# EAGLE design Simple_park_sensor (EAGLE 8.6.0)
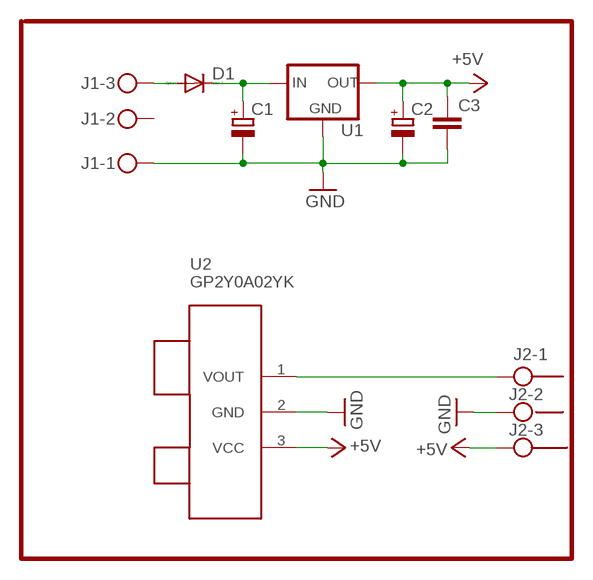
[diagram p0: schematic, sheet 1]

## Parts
C1  CPOL-EUC/6032-28W  [C/6032-28W]
C2  CPOL-EUC/6032-28W  [C/6032-28W]
C3  C-EUC1206  [C1206]
D1  CGRM4002-G  [SOD-123_MINI-SMA]
J1  MKDSN1,5/3-5,08  [MKDSN1,5/3-5,08]
J2  MKDSN1,5/3-5,08  [MKDSN1,5/3-5,08]
U1  78XXL  [78XXL]
U2  GP2Y0A02YK  [GP2Y0A02YK]

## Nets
+5V: C2.+ C3.1 J2.3 U1.OUT U2.3(VCC)
GND: C1.- C2.- C3.2 J1.1 J2.2 U1.GND U2.2(GND)
N$1: C1.+ D1.C U1.IN
N$2: D1.A J1.3
N$3: J2.1 U2.1(VOUT)
Unconnected: J1.2

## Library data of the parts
C1 C2 = rcl:CPOL-EU: POLARIZED CAPACITOR, European symbol
C3 = rcl:C-EU: CAPACITOR, European symbol
D1 = diode:CGRM400*-G: Molded plasitc,JEDEC SOD-123/Mini SMA
J1 J2 = con-phoenix-508:MKDSN1,5/3-5,08: MKDSN 1,5/ 3-5,08 Printklemme Nennstrom: 13,5 A Nennspannung: 250 V Rastermaß: 5,08 mm Polzahl: 3 Anschlussart: Schraubanschluss Montage: Löten Anschlussrichtung Leiter/Platine: 0 ° Artikelnummer: 1729131 Source: http://eshop.phoenixcontact.com .. 1729131.pdf
U1 = v-reg:78XXL: VOLTAGE REGULATOR
U2 = sharp:GP2Y0A02YK

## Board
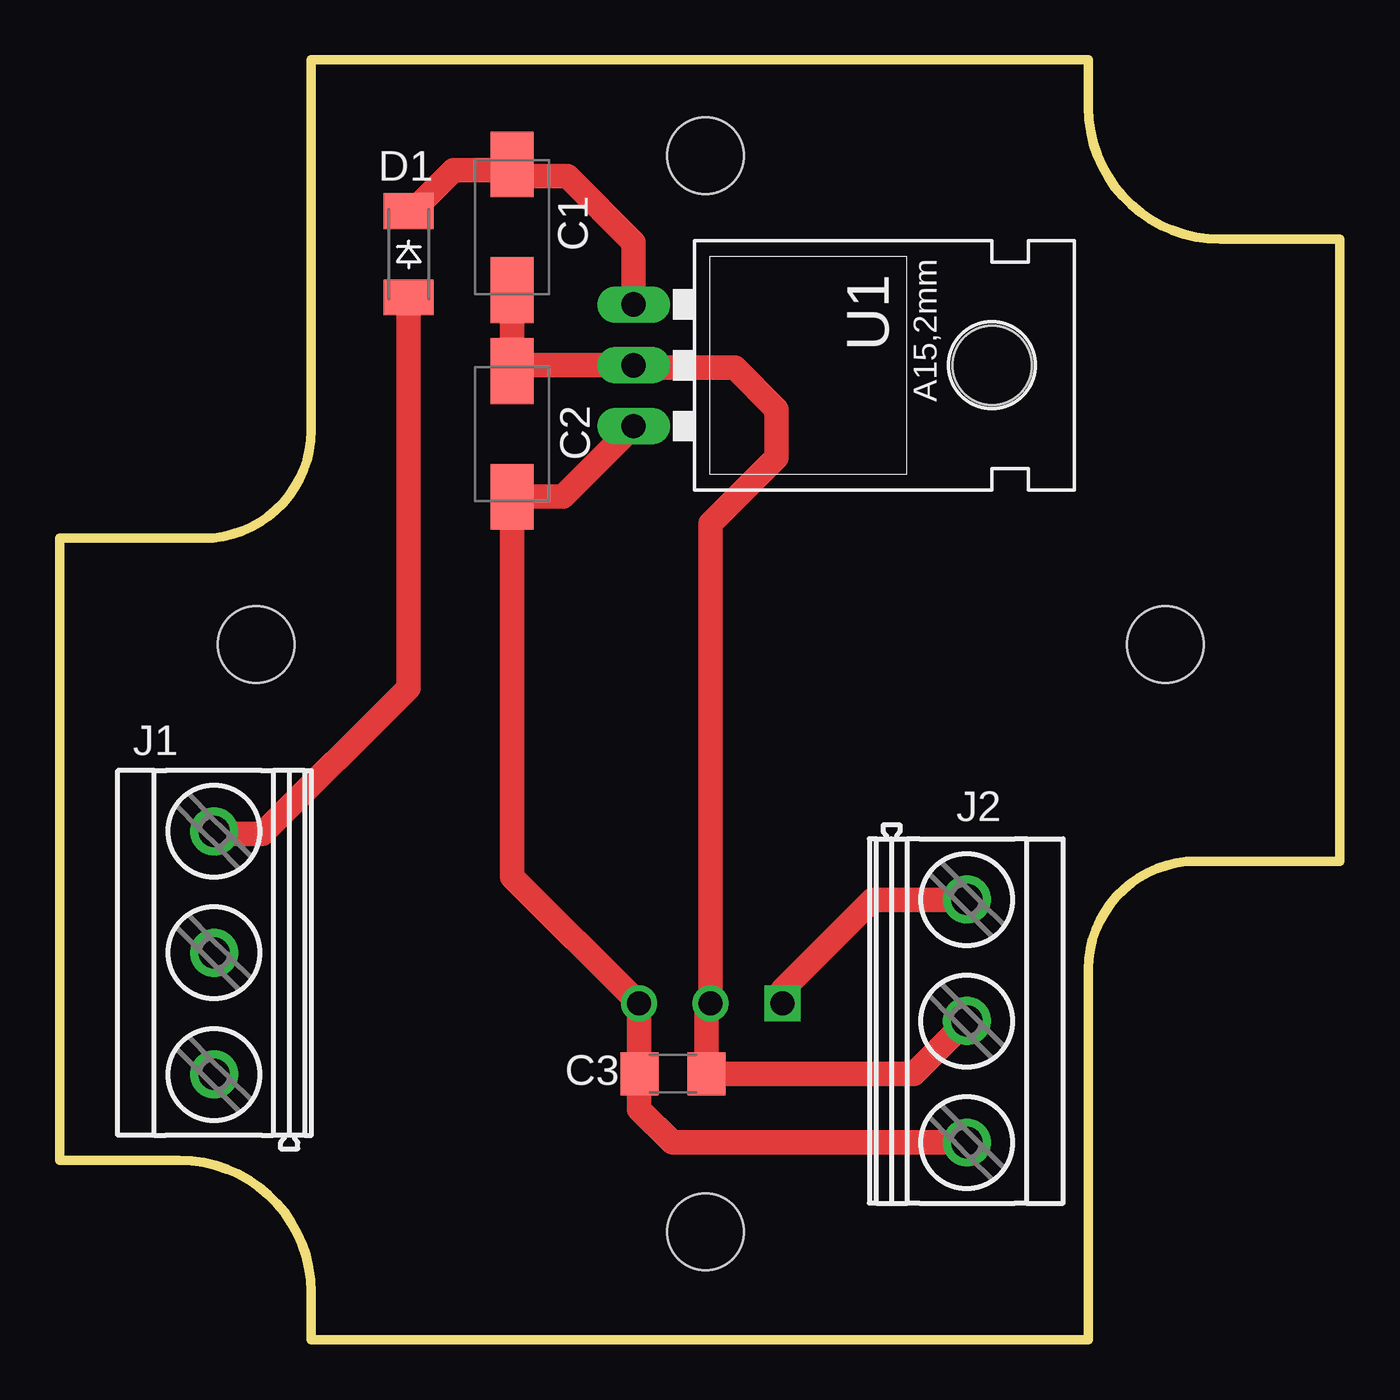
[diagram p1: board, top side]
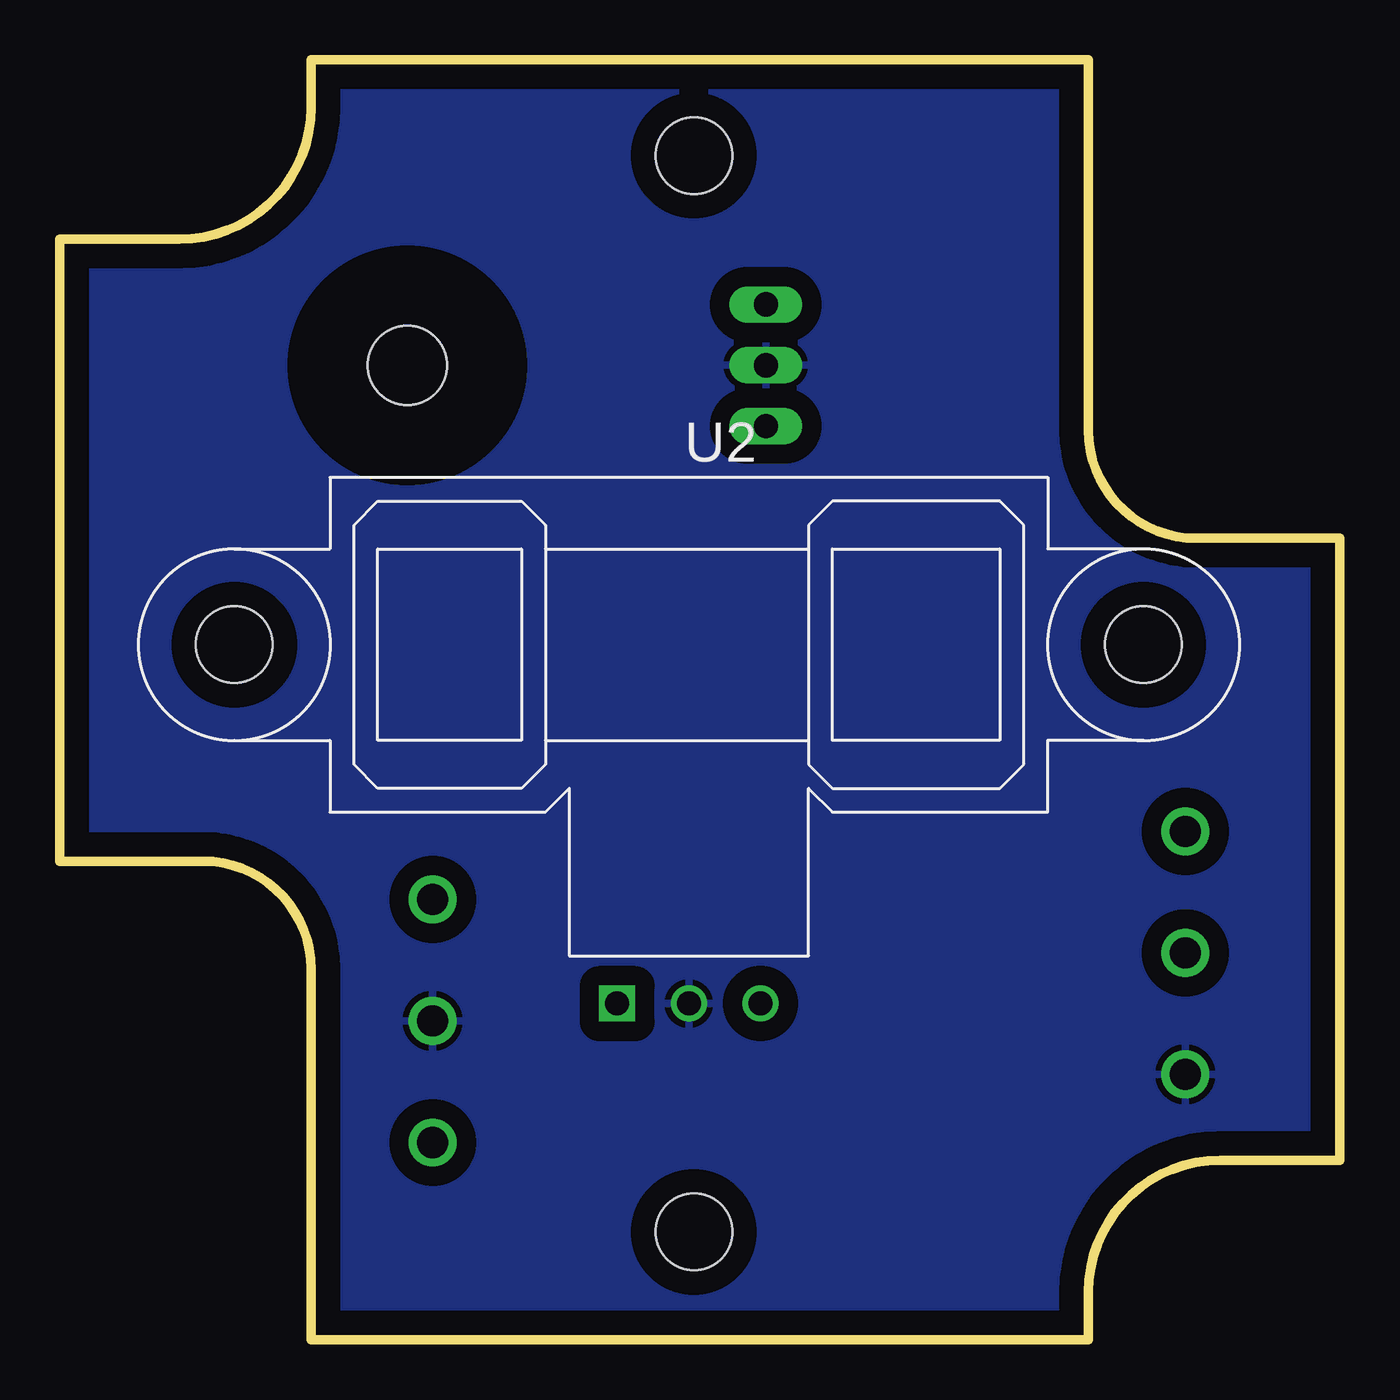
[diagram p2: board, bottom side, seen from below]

Size 53.5 x 53.5 mm. Coordinates in mm from the lower left corner, seen from the top.
Outline: 0,7.5 0,33.5 6,33.5 arc90 10.5,38 10.5,53.5 43,53.5 43,51.5 arc90 48.5,46 53.5,46 53.5,20 47.5,20 arc90 43,15.5 43,0 10.5,0 10.5,2 arc90 5,7.5 0,7.5
Copper layers (1*16): Top 0.035mm / dielectric 1.5mm / Bottom 0.035mm
Design rules "default": minimum track width 10mil, minimum drill 24mil, track to track 8mil, track to pad 8mil, pad to pad 8mil, via to via 8mil, smd to smd 8mil, copper to edge 40mil, drill to drill 8mil, minimum pad ring 10mil, minimum via ring 8mil, stop-mask expansion 4mil, vias tented up to drill 0mil, thermal gap 10mil
Holes 3.2 mm at 27,4.5 27,49.5

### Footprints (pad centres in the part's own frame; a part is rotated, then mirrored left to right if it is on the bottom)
C/6032-28W = smd 2.75 x 1.8: + 2.625,0; - -2.625,0
C1206 = smd 1.6 x 1.8: 1 -1.4,0; 2 1.4,0
SOD-123_MINI-SMA = smd 1.5 x 2.1: A 1.8,0; C -1.8,0
MKDSN1,5/3-5,08 = drill 1.3 pad 2: 1 -7.641,0.025; 2 -2.561,0.025; 3 2.519,0.025
78XXL = drill 1.016 long: GND 0,-3.81; IN -2.54,-3.81; OUT 2.54,-3.81 | hole 3.302: 0,11.176
GP2Y0A02YK = drill 1 square: 1 16,-15 | drill 1: 2 19,-15; 3 22,-15 | hole 3.2: 0,0; 38,0

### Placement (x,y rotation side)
C1  18.91,46.5 90 top
C2  18.91,37.86 270 top
C3  25.64,11.12 0 top
D1  14.58,45.37 270 top
J1  6.47,18.73 90 top
J2  37.89,10.76 270 top
U1  27.79,40.73 270 top
U2  46.21,29.05 0 bottom

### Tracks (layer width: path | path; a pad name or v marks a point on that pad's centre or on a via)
+5V
  Top 1.016: U1.OUT 21.03,35.23 C2.+ 18.91,19.35 U2.3 24.2,11.15 C3.1 24.21,11.1 24.21,9.63 25.6,8.24 J2.3
GND
  Top 1.016: C1.- C2.- 19.15,40.73 U1.GND 24.09,40.63 28.21,40.63 29.96,38.88 29.96,36.88 27.2,34.12 U2.2 27.04,13.88 C3.2 35.71,11.12 J2.2
  pour Bottom (isolate 0.813): -0.28,53.63 53.97,53.63 53.97,-0.37 -0.28,-0.37
N$1
  Top 1.016: D1.C 14.75,47.17 16.46,48.88 18.65,48.88 C1.+ 18.91,48.63 21.21,48.63 23.98,45.86 U1.IN
N$2
  Top 1.016: D1.A 14.58,27.25 8.46,21.13 6.57,21.13 J1.3
N$3
  Top 1.016: U2.1 30.2,14.62 33.97,18.38 37.89,18.38 J2.1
